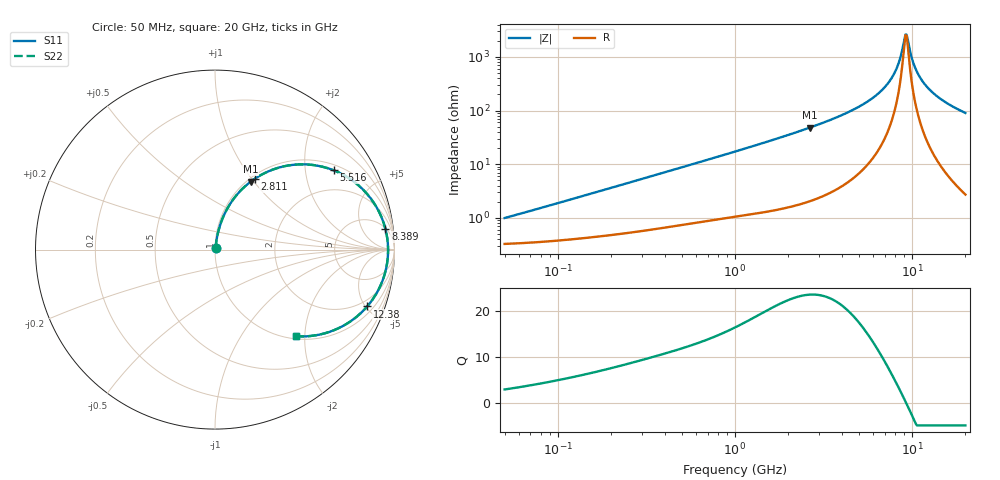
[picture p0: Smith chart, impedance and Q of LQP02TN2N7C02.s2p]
!Murata Part Number: LQP02TN2N7C02
!These Parameters are Measured in Series Mode Connection
!  o--[Z]--o
!Port1  Port2
!  o-------o
!Freq. Start=50[MHz] Stop=20[GHz], 401[Steps]
# Hz S RI R 50
!Freq.(Hz) S11(Real) S11(Imag) S21(Real) S21(Imag) S12(Real) S12(Imag) S22(Real) S22(Imag)
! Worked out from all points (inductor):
!   401 points, 50 MHz to 20 GHz, reference 50 ohm
!   read as one part in series: L = 2.96 nH near 53.09 MHz
!   highest Q = 23.6 at 2.647 GHz (marker M1), where L = 2.89 nH
!   self-resonance near 9.178 GHz
!   S11 on the Smith chart (normalised r, x): 50 MHz: 1.01, +0.02; 2.811 GHz: 1.04, +1.03; 5.516 GHz: 1.18, +2.84; 8.389 GHz: 5, +15; 12.38 GHz: 1.46, -5.13; 20 GHz: 1.05, -1.81
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5e7  0.00333 0.0093  0.9967 -0.0093  0.9967 -0.0093  0.00333 0.0093
1.364002e8  0.00473 0.0246  0.9953 -0.0246  0.9953 -0.0246  0.00473 0.0246
3.721004e8  0.0105 0.0643  0.9895 -0.0643  0.9895 -0.0643  0.0105 0.0643
1e9  0.0381 0.1633  0.9619 -0.1633  0.9619 -0.1633  0.0381 0.1633
1.740566e9  0.0945 0.2701  0.9055 -0.2701  0.9055 -0.2701  0.0945 0.2701
2.647493e9  0.1984 0.3782  0.8016 -0.3782  0.8016 -0.3782  0.1984 0.3782
2.728004e9  0.2093 0.3862  0.7907 -0.3862  0.7907 -0.3862  0.2093 0.3862
2.810964e9  0.2207 0.3941  0.7793 -0.3941  0.7793 -0.3941  0.2207 0.3941
4.212059e9  0.4424 0.473  0.5576 -0.473  0.5576 -0.473  0.4424 0.473
5.515528e9  0.6603 0.4422  0.3397 -0.4422  0.3397 -0.4422  0.6603 0.4422
6.503449e9  0.8001 0.3576  0.1999 -0.3576  0.1999 -0.3576  0.8001 0.3576
7.442007e9  0.8955 0.244  0.1045 -0.244  0.1045 -0.244  0.8955 0.244
7.901521e9  0.927 0.1821  0.073 -0.1821  0.073 -0.1821  0.927 0.1821
8.389408e9  0.9495 0.1148  0.0505 -0.1148  0.0505 -0.1148  0.9495 0.1148
9.041845e9  0.9634 0.026  0.0366 -0.026  0.0366 -0.026  0.9634 0.026
9.316812e9  0.9643 -0.0102  0.0357 0.0102  0.0357 0.0102  0.9643 -0.0102
1.004137e10  0.9545 -0.0999  0.0455 0.0999  0.0455 0.0999  0.9545 -0.0999
1.050288e10  0.9408 -0.1518  0.0592 0.1518  0.0592 0.1518  0.9408 -0.1518
1.131968e10  0.906 -0.2327  0.094 0.2327  0.094 0.2327  0.906 -0.2327
1.238412e10  0.8481 -0.3166  0.1519 0.3166  0.1519 0.3166  0.8481 -0.3166
1.527346e10  0.6743 -0.4444  0.3257 0.4444  0.3257 0.4444  0.6743 -0.4444
2e10  0.4506 -0.4828  0.5494 0.4828  0.5494 0.4828  0.4506 -0.4828
